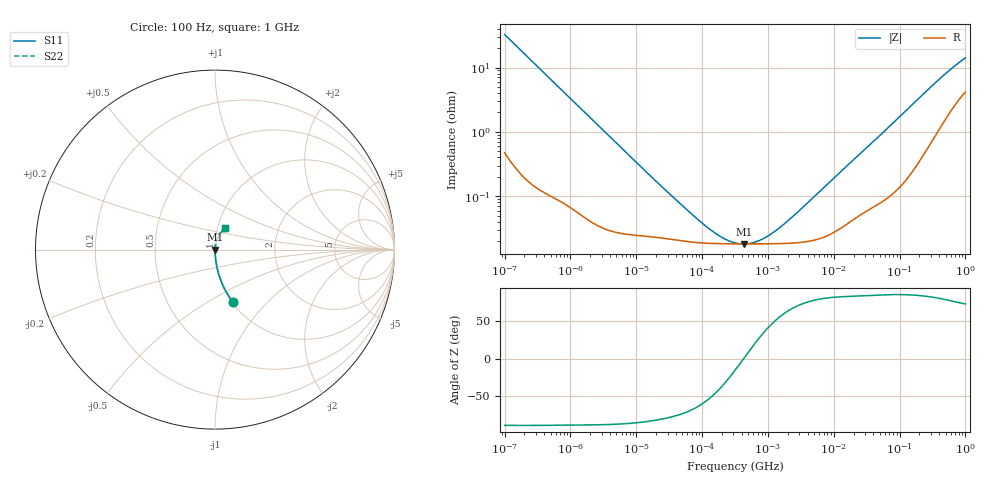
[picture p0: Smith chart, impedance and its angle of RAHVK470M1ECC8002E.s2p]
! RAHVK470M1ECC8002E  S-PARAMETER MODEL  (AEC-Q200 qualified)
! Model Generated by ELNA Corporation (http://www.ty-top.com)
! Version 1.0
! ELNA Control No.201026
! Copyright (c) 2020 ELNA CO.,LTD. All Rights Reserved.
! Products Name : CONDUCTIVE POLYMER HYBRID ALUMINUM ELECTROLYTIC CAPACITORS
! Characteristics :
!  Capacitance  :  47uF  ,  Rated voltage  :  16V
!  Operating Temp. Range  :  -55 to +125 degC  ,  Endurance  :  4000hr at 125 degC
!  Dimension D  :  5mm  ,  Dimension L  :  5.8mm
! Frequency Range : 100Hz - 1GHz
! External Node Assignments :
!  1  o---| |---o  2
# MHz S RI R 50
!Freq[MHz].  S11 Real  S11 Imag  S21 Real  S21 Imag  S12 Real  S12 Imag  S22 Real  S22 Imag
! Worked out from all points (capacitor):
!   401 points, 100 Hz to 1 GHz, reference 50 ohm
!   read as one part in series: C = 48.8 uF near 108 Hz
!   lowest |Z| = 18.2 mohm at 436.5 kHz (marker M1)
!   series resonance near 428.6 kHz, so ESL is about 2.8 nH
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0.0001  0.0996 -0.2922  0.9004 0.2922  0.9004 0.2922  0.0996 -0.2922
0.000113  0.0801 -0.2648  0.9199 0.2648  0.9199 0.2648  0.0801 -0.2648
0.000162  0.041 -0.1924  0.959 0.1924  0.959 0.1924  0.041 -0.1924
0.000309  0.0123 -0.1043  0.9877 0.1043  0.9877 0.1043  0.0123 -0.1043
0.000613  0.00375 -0.0533  0.9963 0.0533  0.9963 0.0533  0.00375 -0.0533
0.001488  0.000995 -0.0222  0.999 0.0222  0.999 0.0222  0.000995 -0.0222
0.022131  0.000229 -0.00153  0.9998 0.00153  0.9998 0.00153  0.000229 -0.00153
0.06569  0.000195 -0.000521  0.9998 0.000521  0.9998 0.000521  0.000195 -0.000521
0.12517  0.000185 -0.000258  0.9998 0.000258  0.9998 0.000258  0.000185 -0.000258
0.203002  0.000183 -0.000135  0.9998 0.000135  0.9998 0.000135  0.000183 -0.000135
0.316228  0.000182 -5.11e-05  0.9998 5.11e-05  0.9998 5.11e-05  0.000182 -5.11e-05
0.436516  0.000181 3.08e-06  0.9998 -3.08e-06  0.9998 -3.08e-06  0.000181 3.08e-06
0.533949  0.000181 3.68e-05  0.9998 -3.68e-05  0.9998 -3.68e-05  0.000181 3.68e-05
0.679986  0.000182 7.93e-05  0.9998 -7.93e-05  0.9998 -7.93e-05  0.000182 7.93e-05
1.102808  0.000182 0.000181  0.9998 -0.000181  0.9998 -0.000181  0.000182 0.000181
1.938653  0.000185 0.000356  0.9998 -0.000356  0.9998 -0.000356  0.000185 0.000356
4.704354  0.000205 0.000898  0.9998 -0.000898  0.9998 -0.000898  0.000205 0.000898
69.9842  0.00113 0.0121  0.9989 -0.0121  0.9989 -0.0121  0.00113 0.0121
176.8072  0.00375 0.0298  0.9962 -0.0298  0.9962 -0.0298  0.00375 0.0298
395.8221  0.0146 0.0626  0.9854 -0.0626  0.9854 -0.0626  0.0146 0.0626
695.825  0.0353 0.0973  0.9647 -0.0973  0.9647 -0.0973  0.0353 0.0973
1000  0.0558 0.1226  0.9442 -0.1226  0.9442 -0.1226  0.0558 0.1226
